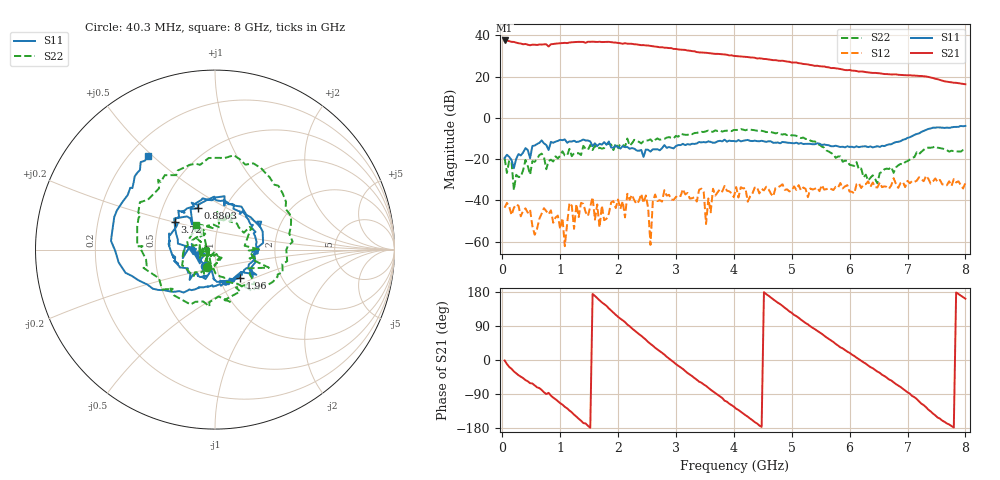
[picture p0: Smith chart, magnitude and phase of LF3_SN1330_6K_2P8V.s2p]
! VC=2.8V I=23.7mA
# HZ S DB R 50.00
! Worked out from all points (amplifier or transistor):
!   200 points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, 40.3 MHz to 8 GHz, reference 50 ohm
!   highest |S21| = 37.6 dB at 40.3 MHz (marker M1)
!   |S21| within 3 dB of that: start of sweep to 2.647 GHz
!   unconditionally stable (mu >= 1): start of sweep to 2.158 GHz; 2.169 GHz to 2.793 GHz; 4.201 GHz to end of sweep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
!   at 1.36 GHz: K = 1.08, MAG = 37.3 dB, |S12| = -41.1 dB
!   at 4.04 GHz: K = 0.96, MSG = 31.7 dB, |S12| = -33.5 dB
!   at 8 GHz: K = 1.75, MAG = 18.9 dB, |S12| = -31.5 dB
!   S11 on the Smith chart (normalised r, x): 40.3 MHz: 0.88, -0.16; 880.3 MHz: 0.75, +0.37; 1.96 GHz: 1.25, -0.41; 3.72 GHz: 0.61, +0.20; 8 GHz: 0.27, +0.49
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4.02985e7  -19.40 -122.2  37.58 -1.3  -43.53 67.7  -19.40 -116.2
1.202955e8  -18.86 -137.6  37.26 -18.4  -43.01 1.3  -20.52 -102.6
2.802895e8  -17.48 166.2  36.23 -40.1  -42.55 106.5  -28.61 165.9
8.80267e8  -12.04 112.9  35.86 -99.4  -50.79 105.7  -21.10 151.8
1.160256e9  -11.38 78.9  36.60 -133.3  -41.22 -50.0  -14.98 125.7
1.400248e9  -10.42 31.2  36.85 -166.6  -41.67 14.9  -13.53 86.6
1.680237e9  -12.51 -16.7  36.97 157.5  -53.07 45.8  -14.43 49.9
1.960226e9  -13.54 -48.3  36.54 119.2  -43.66 -19.8  -12.25 0.3
2.240216e9  -14.57 -73.8  35.95 83.4  -37.25 -29.2  -12.31 -36.0
2.520206e9  -15.44 -115.2  35.12 47.5  -43.78 -44.4  -10.85 -79.2
2.720198e9  -15.69 -126.3  34.26 23.4  -39.86 -44.2  -10.56 -102.8
2.92019e9  -14.45 -145.4  33.87 -1.0  -39.61 -86.9  -9.62 -138.9
3.240178e9  -12.94 -169.4  32.62 -38.6  -39.11 -113.4  -7.58 178.5
3.72016e9  -11.33 145.1  31.09 -91.8  -36.02 -168.8  -6.31 128.7
4.040148e9  -11.43 115.8  30.01 -128.5  -33.48 -172.7  -5.83 88.8
4.560129e9  -11.58 73.0  28.56 173.6  -33.33 141.8  -6.86 30.0
4.960114e9  -12.06 41.7  27.25 128.1  -35.61 115.7  -8.01 -18.5
5.360099e9  -12.75 7.0  25.52 85.0  -34.70 64.4  -11.39 -51.0
6.000075e9  -14.04 -44.8  23.27 18.8  -35.73 28.6  -22.71 -129.5
6.68005e9  -12.84 -113.4  21.20 -51.4  -34.32 5.3  -24.73 -76.0
7.360024e9  -5.33 -172.5  19.91 -130.9  -29.47 -94.7  -14.39 -137.7
8e9  -3.87 125.4  16.35 161.8  -31.52 -164.9  -15.28 127.9
